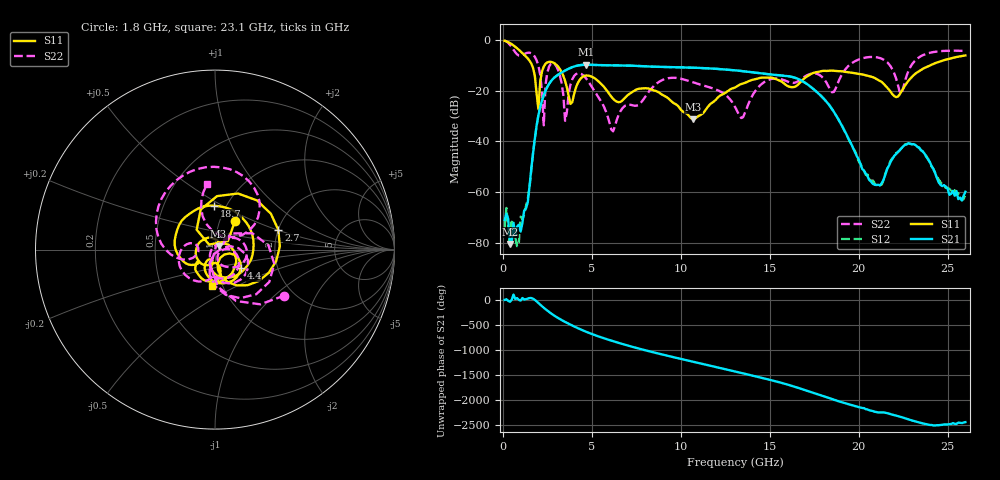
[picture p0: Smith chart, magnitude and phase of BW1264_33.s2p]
!Keysight Technologies,N5245B,MY57181159,A.13.60.06
!Date: Friday, December 18, 2020 23:53:43
!Correction: S11(Full 2 Port(1,2))
!S21(Full 2 Port(1,2))
!S12(Full 2 Port(1,2))
!S22(Full 2 Port(1,2))
!S2P File: Measurements: S11, S21, S12, S22:
# Hz S  dB  R 50
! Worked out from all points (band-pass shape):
!   260 points, 100 MHz to 26 GHz, reference 50 ohm
!   highest |S21| = -9.80 dB at 4.7 GHz (marker M1); lowest = -80.6 dB at 400 MHz (marker M2)
!   |S21| within 3 dB of the highest: 3.322 GHz to 14.07 GHz (10.74 GHz wide, 124 % of centre)
!   lowest |S11| = -31.3 dB at 10.7 GHz (marker M3), VSWR 1.06, Z = 52 + j1.94 ohm
!   |S11| at or under -10 dB: 1.638 GHz to 2.347 GHz (708.4 MHz wide, 35.6 % of centre); 3.036 GHz to 24.03 GHz (20.99 GHz wide, 155 % of centre)
!   |S22| runs from -36.1 to -0.2 dB; largest |S21 - S12| = 0.00073
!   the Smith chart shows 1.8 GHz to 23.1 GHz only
!   S11 on the Smith chart (normalised r, x): 1.8 GHz: 1.18, +0.39; 2.7 GHz: 2.01, +0.51; 4.4 GHz: 1.30, -0.28; 18.7 GHz: 0.88, +0.46; 23.1 GHz: 0.89, -0.38
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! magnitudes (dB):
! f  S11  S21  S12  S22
! 100 MHz  -0.3  -71.2  -74.3  -0.2
! 400 MHz  -1.3  -80.6  -80.9  -1.9
! 900 MHz  -3.9  -72.9  -80.1  -6.1
! 1.8 GHz  -14.2  -38.9  -38.7  -6.7
! 2 GHz  -27.3  -29.7  -29.7  -10.2
! 2.3 GHz  -10.5  -21.8  -21.8  -33.7
! 2.7 GHz  -8.6  -16.3  -16.3  -9.4
! 3.5 GHz  -16.2  -12.1  -12.1  -31.9
! 4.4 GHz  -15.1  -9.9  -9.9  -13.4
! 4.5 GHz  -14.5  -9.8  -9.8  -13.9
! 4.7 GHz  -14.0  -9.8  -9.8  -15.4
! 6.2 GHz  -23.2  -10.0  -10.0  -36.1
! 8.8 GHz  -20.9  -10.6  -10.6  -16.4
! 10.7 GHz  -31.3  -11.0  -10.9  -16.7
! 13.1 GHz  -18.6  -12.0  -12.0  -27.0
! 17.4 GHz  -13.2  -19.0  -19.0  -13.2
! 18.7 GHz  -12.2  -29.4  -29.4  -19.3
! 20.8 GHz  -14.7  -56.8  -55.5  -6.7
! 21.7 GHz  -19.6  -49.7  -49.2  -9.5
! 22.4 GHz  -20.4  -42.8  -42.7  -21.3
! 23.1 GHz  -13.9  -41.1  -41.4  -8.7
! 26 GHz  -6.1  -59.9  -60.8  -4.3
